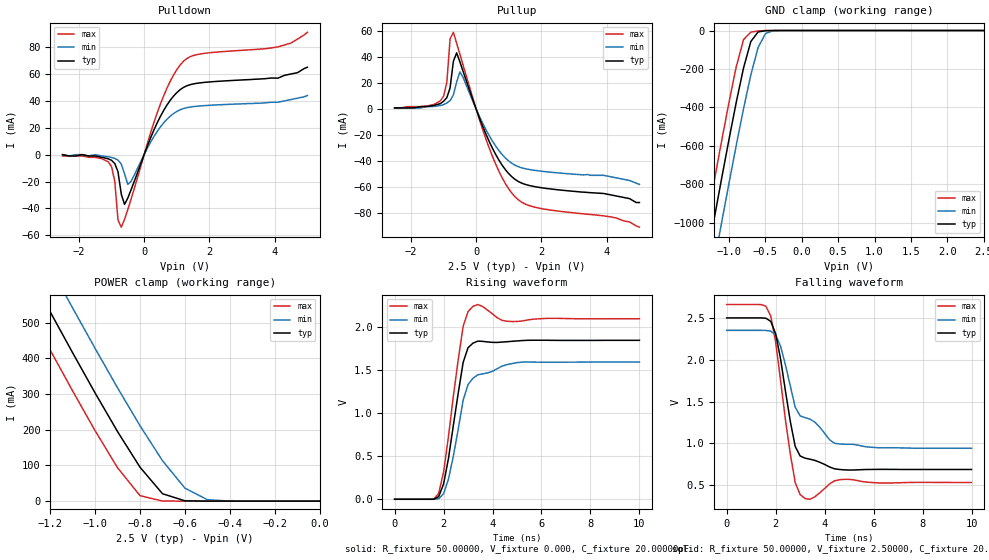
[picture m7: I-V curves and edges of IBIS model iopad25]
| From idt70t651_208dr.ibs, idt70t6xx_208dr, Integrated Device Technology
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|   Model iopad25
[Model]   iopad25
Model_type   I/O
Polarity   Non-Inverting
Enable   Active-Low
Vinl =  0.70000V
Vinh =  1.70000V
Vmeas =  1.25000V
C_comp   4.50000pF   4.50000pF   4.50000pF
[Temperature Range]   25.00000   100.00000   -40.00000
[Voltage Range]   2.50000V   2.30000V   2.70000V
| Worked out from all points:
|   slope of the pulldown table from 0 to 0.375 V, typ, clamps not added: 16.8 ohm
|   slope of the pullup table from 0 to 0.375 V, typ, clamps not added: 15.9 ohm
|   GND clamp passes 1 mA (typ) near -0.50 V on its own axis
|   POWER clamp passes 1 mA (typ) near -0.60 V on its own axis
|   rising waveform, R_fixture 50.00000, V_fixture 0.000, C_fixture 20.00000pF: 20-80 % time 607ps typ, 673ps min, 577ps max; typ from 0 V to 1.85 V
|   falling waveform, R_fixture 50.00000, V_fixture 2.50000, C_fixture 20.00000pF: 20-80 % time 626ps typ, 1.42ns min, 572ps max; typ from 2.5 V to 0.689 V
[Pulldown]
| voltage   I(typ)   I(min)   I(max)
-2.5V     0A         0A         -1mA
-1.1V     -3.1mA     -1.6mA     -5.4mA
-1V       -4.2mA     -2.1mA     -8.8mA
-900mV    -6.6mA     -2.8mA     -19.8mA
-800mV    -12.8mA    -4.1mA     -48.76mA
-700mV    -29.43mA   -7mA       -53.96mA
-600mV    -37.03mA   -14.17mA   -48.13mA
-500mV    -32.29mA   -22.11mA   -40.89mA
500mV     28.49mA    20.63mA    37.7mA
1.2V      49.93mA    34.24mA    69.32mA
4.1V      56.9mA     39mA       80.2mA
5V        65mA       44mA       91mA
[Pullup]
| voltage   I(typ)   I(min)   I(max)
-2.5V     1mA        1mA        1mA
-1.1V     4.3mA      2.9mA      6.4mA
-900mV    8.9mA      4.8mA      20.66mA
-800mV    16.52mA    6.6mA      54.26mA
-700mV    36.86mA    11mA       59.33mA
-600mV    43.46mA    20.89mA    50.96mA
-500mV    36.57mA    28.78mA    42.4mA
400mV     -24.99mA   -20.52mA   -30.09mA
800mV     -43.39mA   -35.12mA   -53.17mA
1.2V      -54.33mA   -43.34mA   -67.83mA
1.8V      -59.77mA   -47.2mA    -75.63mA
5V        -72mA      -58mA      -91mA
[GND_clamp]
| voltage   I(typ)   I(min)   I(max)
-2.5V     -3.74A     -3.961A    -3.553A
-1.4V     -1.389A    -1.618A    -1.194A
-1.3V     -1.179A    -1.409A    -984.4mA
-1.2V     -972.3mA   -1.201A    -776.5mA
-1.1V     -767.3mA   -996.6mA   -571.8mA
-900mV    -372.8mA   -596.6mA   -188mA
-800mV    -194.3mA   -406.4mA   -47.16mA
-700mV    -57.22mA   -230.7mA   -8.4mA
-600mV    -7.393mA   -88.33mA   -2.169mA
-500mV    -1.009mA   -16.09mA   -229.2uA
-400mV    -92.71uA   -1.476mA   -9.663uA
2.5V      510.3pA    625.2nA    1.837pA
[POWER_clamp]
| voltage   I(typ)   I(min)   I(max)
-2.5V     2.074A     2.195A     1.972A
-1.4V     762.2mA    887.1mA    656mA
-1.3V     645.3mA    770.5mA    538.7mA
-1.2V     529.4mA    654.8mA    422.5mA
-1.1V     414.9mA    540.2mA    308mA
-1V       302.5mA    427.3mA    196.9mA
-900mV    194.4mA    316.8mA    93.14mA
-800mV    94.88mA    210.9mA    15.33mA
-700mV    20.78mA    113.2mA    204uA
-600mV    865.9uA    36.42mA    1.94uA
-500mV    23.06uA    3.99mA     31.75nA
0V        510.3pA    46.37nA    1.886pA
[Ramp]
| variable   typ   min   max
dV/dt_r   1.11300/0.34369n   0.96060/0.43779n   1.26420/0.27148n
dV/dt_f   1.08936/0.31359n   0.87954/0.39756n   1.27392/0.24899n
R_load = 50.00000
[Rising Waveform]
R_fixture = 50.00000
V_fixture = 0.000
C_fixture = 20.00000pF
R_dut = 0.19600
L_dut = 13.10000nH
C_dut = 1.92000pF
| time   V(typ)   V(min)   V(max)
0s        0V         0V         0V
1.6ns     202.8uV    -879.7uV   1.405mV
1.8ns     30.68mV    6.028mV    68.03mV
2ns       177.6mV    64.28mV    315.4mV
2.2ns     474.6mV    233.5mV    730.6mV
2.8ns     1.593V     1.154V     2.013V
3ns       1.764V     1.335V     2.184V
3.2ns     1.817V     1.409V     2.245V
4.6ns     1.834V     1.567V     2.072V
10ns      1.85V      1.597V     2.101V
[Falling Waveform]
R_fixture = 50.00000
V_fixture = 2.50000
C_fixture = 20.00000pF
R_dut = 0.19600
L_dut = 13.10000nH
C_dut = 1.92000pF
| time   V(typ)   V(min)   V(max)
0s        2.5V       2.351V     2.66V
1.4ns     2.5V       2.351V     2.659V
1.8ns     2.458V     2.342V     2.524V
2ns       2.311V     2.297V     2.212V
2.2ns     2.011V     2.162V     1.756V
2.6ns     1.26V      1.685V     871.6mV
2.8ns     963.4mV    1.432V     532.2mV
3.2ns     824.2mV    1.308V     342.3mV
4.4ns     697.1mV    1.002V     552.9mV
10ns      689mV      942.3mV    533.3mV
